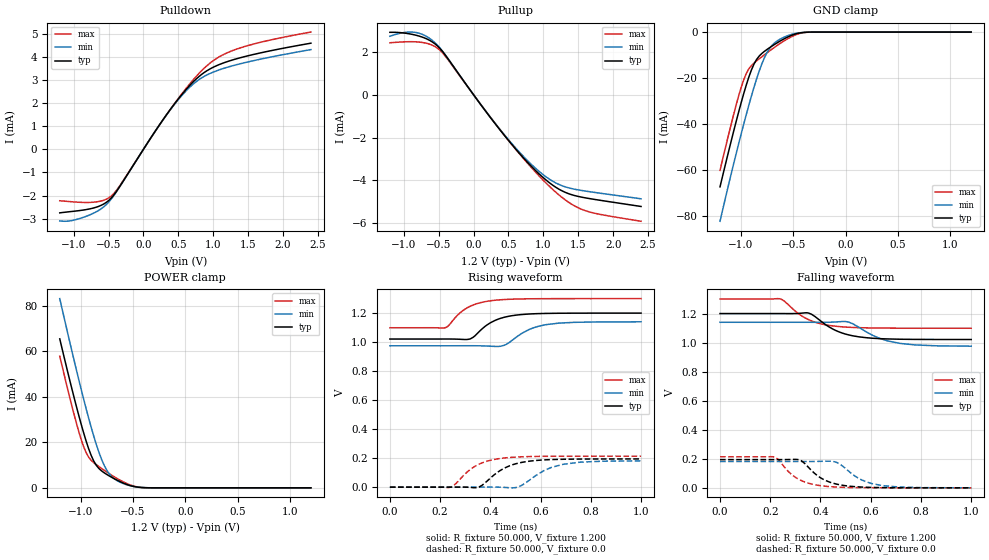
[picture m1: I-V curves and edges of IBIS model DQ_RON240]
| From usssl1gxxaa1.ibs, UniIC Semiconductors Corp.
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|   Model DQ_RON240
[Model] DQ_RON240
Model_type I/O
Vinl =  0.500V
Vinh =  0.700V
Vmeas =  0.600V
Rref =  50.000
Vref =  0.600V
C_comp   1.373pF   1.353pF   1.403pF
[Model Spec]
Vinh   0.700V   0.670V   0.750V
Vinl   0.500V   0.470V   0.550V
Vmeas   0.600V   0.570V   0.650V
Vref   0.600V   0.570V   0.650V
Rref   50.000   NA   NA
[Temperature Range]   25.000   0.125k   -40.000
[Voltage Range]   1.200V   1.140V   1.300V
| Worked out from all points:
|   slope of the pulldown table from 0 to 0.18 V, typ, clamps not added: 216 ohm
|   slope of the pullup table from 0 to 0.18 V, typ, clamps not added: 226 ohm
|   GND clamp passes 1 mA (typ) near -0.49 V on its own axis
|   POWER clamp passes 1 mA (typ) near -0.53 V on its own axis
|   rising waveform, R_fixture 50.000, V_fixture 1.200: 20-80 % time 94.3ps typ, 104ps min, 91.5ps max; typ from 1.02 V to 1.2 V
|   rising waveform, R_fixture 50.000, V_fixture 0.0: 20-80 % time 105ps typ, 116ps min, 99.8ps max; typ from 0 V to 0.194 V
|   falling waveform, R_fixture 50.000, V_fixture 1.200: 20-80 % time 114ps typ, 126ps min, 109ps max; typ from 1.2 V to 1.02 V
|   falling waveform, R_fixture 50.000, V_fixture 0.0: 20-80 % time 93.3ps typ, 100ps min, 90.1ps max; typ from 0.195 V to 0 V
[Pulldown]
|Voltage   I(typ)   I(min)   I(max)
-1.2V     -2.75mA    -3.097mA   -2.227mA
-1.015V   -2.686mA   -3.076mA   -2.273mA
-756mV    -2.569mA   -2.82mA    -2.297mA
-571mV    -2.369mA   -2.494mA   -2.206mA
-460mV    -2.102mA   -2.147mA   -2.019mA
-349mV    -1.65mA    -1.664mA   -1.619mA
354mV     1.593mA    1.581mA    1.593mA
613mV     2.591mA    2.531mA    2.639mA
798mV     3.149mA    3.016mA    3.285mA
1.02V     3.574mA    3.359mA    3.872mA
1.279V    3.862mA    3.61mA     4.268mA
2.4V      4.585mA    4.308mA    5.066mA
[Pullup]
|Voltage   I(typ)   I(min)   I(max)
-1.2V     2.921mA    2.737mA    2.433mA
-1.004V   2.89mA     2.908mA    2.474mA
-819mV    2.779mA    2.908mA    2.474mA
-634mV    2.552mA    2.645mA    2.37mA
-486mV    2.179mA    2.203mA    2.097mA
106mV     -472.6uA   -469.2uA   -466.4uA
513mV     -2.182mA   -2.147mA   -2.182mA
846mV     -3.4mA     -3.306mA   -3.462mA
1.142V    -4.24mA    -4.052mA   -4.445mA
1.364V    -4.621mA   -4.347mA   -5.024mA
1.586V    -4.804mA   -4.488mA   -5.395mA
2.4V      -5.216mA   -4.857mA   -5.907mA
[GND_clamp]
|Voltage   I(typ)   I(min)   I(max)
-1.2V     -67.26mA   -82.22mA   -60.1mA
-1.05V    -39.62mA   -53.62mA   -32.4mA
-1V       -31.05mA   -44.64mA   -24.37mA
-950mV    -23.16mA   -36.01mA   -18.1mA
-925mV    -19.62mA   -31.85mA   -16.02mA
-875mV    -13.89mA   -23.97mA   -13.48mA
-800mV    -9.288mA   -13.81mA   -10.72mA
-750mV    -7.535mA   -8.829mA   -8.993mA
-675mV    -5.274mA   -4.578mA   -6.506mA
-525mV    -1.587mA   -1.138mA   -2.208mA
-375mV    -90.13uA   -87.27uA   -132.9uA
1.2V      0A         0A         0A
[POWER_clamp]
|Voltage   I(typ)   I(min)   I(max)
-1.2V     65.51mA    83.21mA    57.91mA
-1.05V    37.38mA    53.57mA    29.99mA
-1V       28.74mA    44.18mA    21.95mA
-950mV    20.85mA    35.16mA    15.65mA
-925mV    17.34mA    30.84mA    13.56mA
-875mV    11.74mA    22.7mA     11.06mA
-800mV    7.436mA    12.47mA    8.502mA
-750mV    5.864mA    7.69mA     6.933mA
-675mV    3.901mA    3.837mA    4.735mA
-525mV    971.5uA    903.1uA    1.25mA
-400mV    85.95uA    125.9uA    91.19uA
1.2V      0A         0A         0A
[Ramp]
| variable   typ   min   max
dV/dt_r   0.117/0.106n   0.109/0.113n   0.128/0.101n
dV/dt_f   0.107/0.114n   98.815m/0.125n   0.121/0.109n
R_load = 50.000
[Rising Waveform]
R_fixture= 50.000
V_fixture= 1.200
V_fixture_min= 1.140
V_fixture_max= 1.300
|time   V(typ)   V(min)   V(max)
0s        1.021V     974.8mV    1.099V
222ps     1.021V     974.8mV    1.1V
281ps     1.019V     975mV      1.204V
321ps     1.023V     975.1mV    1.248V
378ps     1.107V     973.5mV    1.279V
420ps     1.151V     970.1mV    1.289V
456ps     1.172V     978.3mV    1.294V
552ps     1.194V     1.085V     1.299V
621ps     1.198V     1.12V      1.3V
1ns       1.2V       1.14V      1.3V
[Rising Waveform]
R_fixture= 50.000
V_fixture= 0.0
V_fixture_min= 0.0
V_fixture_max= 0.0
|time   V(typ)   V(min)   V(max)
0s        74.14nV    1.299uV    42.63nV
236ps     10.88uV    -832.2nV   -2.163mV
254ps     82.95uV    -5.677uV   11.61mV
321ps     -1.88mV    -686.9nV   123mV
356ps     1.908mV    80.92uV    159.2mV
440ps     115.7mV    -534.1uV   197.9mV
514ps     166.6mV    3.358mV    208.4mV
613ps     187.8mV    113.6mV    212.5mV
691ps     192.3mV    158mV      213.4mV
1ns       194.5mV    181.2mV    213.7mV
[Falling Waveform]
R_fixture= 50.000
V_fixture= 1.200
V_fixture_min= 1.140
V_fixture_max= 1.300
|time   V(typ)   V(min)   V(max)
0s        1.2V       1.14V      1.3V
239ps     1.2V       1.14V      1.302V
317ps     1.202V     1.14V      1.194V
353ps     1.203V     1.14V      1.158V
392ps     1.161V     1.14V      1.134V
459ps     1.085V     1.142V     1.113V
511ps     1.054V     1.142V     1.106V
637ps     1.027V     1.028V     1.1V
717ps     1.023V     994.6mV    1.099V
1ns       1.021V     975.3mV    1.099V
[Falling Waveform]
R_fixture= 50.000
V_fixture= 0.0
V_fixture_min= 0.0
V_fixture_max= 0.0
|time   V(typ)   V(min)   V(max)
0s        194.5mV    181.5mV    213.7mV
216ps     194.4mV    181.5mV    212.4mV
232ps     194.4mV    181.5mV    195.1mV
282ps     195.2mV    181.5mV    96.57mV
317ps     191.8mV    181.3mV    55.61mV
408ps     61.38mV    182.7mV    13.16mV
461ps     26.76mV    177.3mV    5.663mV
561ps     5.536mV    56.97mV    1.155mV
646ps     1.462mV    15.49mV    298.7uV
1ns       5.507uV    64.28uV    1.11uV
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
